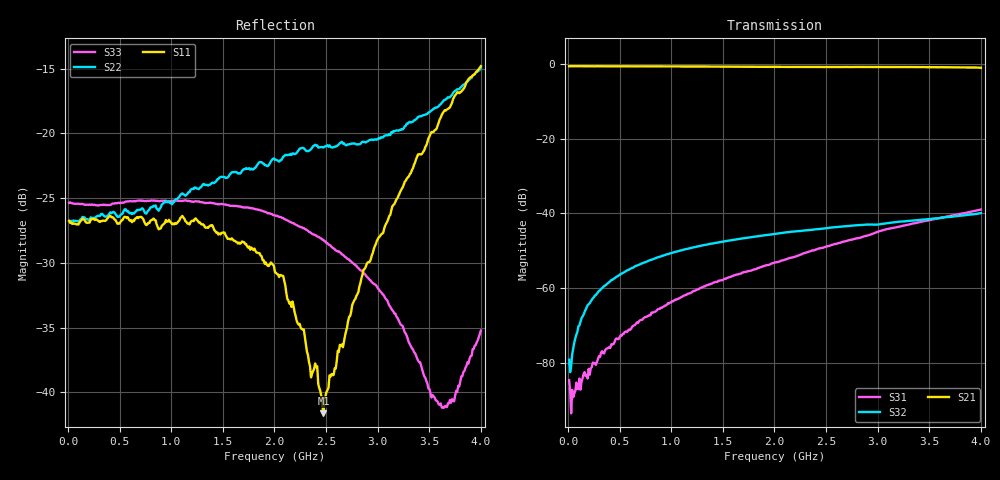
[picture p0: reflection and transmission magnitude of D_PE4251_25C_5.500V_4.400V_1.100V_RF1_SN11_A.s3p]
! Device ID: PE4251_SoldCshunt_081809
! Dir: c:\Test Bench Repositories\Bench_Software_CVI_Version_8\trunk\PSC 4Port_VNA Bench\datalog\4250\TEST\PE4251_SoldCshunt_081809\25C\5p500000\RF1
! Serial: 11
! Insertion: A
! Temp: 25C
! VDD: 5.500
! Control_Hi: 80.000
! Control_Lo: 20.000
! Logic State: RF1
! Port 1: RFC
! Port 2: RF1
! Port 3: RF2
! V1 = 1.10
! V2 = 4.40
! V3 = 1.10
! IDD: 6.772010e-05
! FILE NAME
! DATE 08/18/09  20:15
! CORRECTED  DATA
#  Hz  S  RI  R  50.00
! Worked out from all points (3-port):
!   401 points, 10 MHz to 4 GHz, reference 50 ohm
!   strongest paths, dB at 10 MHz, 1.008 GHz, 2.005 GHz, 3.002 GHz, 4 GHz:
!     S21: -0.6, -0.6, -0.7, -0.7, -1.0
!     S32: -79.2, -50.6, -45.5, -43.0, -39.9
!     S31: -84.7, -63.5, -53.1, -44.9, -39.0
!   lowest |S11| = -41.6 dB at 2.474 GHz (marker M1), VSWR 1.02, Z = 49.9 - j0.828 ohm
!   |S11| at or under -10 dB: start of sweep to end of sweep
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1e7  0.046 -4.05e-05  0.9371 -0.00367  3.37e-05 -4.18e-05
     0.9379 -0.00443  0.0459 5.96e-05  1.15e-05 1.23e-05
     -7.24e-06 -5.79e-05  0.000109 5.09e-06  0.0539 -0.000166
9.9775e7  0.0445 -0.000588  0.9389 -0.0344  2.22e-05 -3.6e-05
          0.9384 -0.0345  0.0457 -0.000485  4.19e-05 0.000299
          9.14e-06 -4.32e-05  3.49e-05 0.000305  0.0535 -0.000366
1.8955e8  0.0452 0.000221  0.9366 -0.0643  -5.5e-06 -7.37e-05
          0.9356 -0.064  0.0466 -0.000106  5.89e-05 0.000574
          1.03e-05 -6.05e-05  5.76e-05 0.000586  0.053 -0.000928
5.0875e8  0.0453 -0.00476  0.9205 -0.1672  -0.000149 -0.000168
          0.9209 -0.1668  0.0483 -0.00367  0.00015 0.00152
          -0.000153 -0.000175  0.000152 0.00153  0.0537 -0.00501
1.137175e9  0.0429 -0.0161  0.8588 -0.3606  -0.000771 -0.00025
            0.859 -0.3591  0.0548 -0.0175  0.000581 0.00326
            -0.000772 -0.000232  0.000574 0.00326  0.0547 -0.00713
2.005e9  0.0263 -0.0126  0.7173 -0.5776  -0.00218 -0.000168
         0.7173 -0.5775  0.0692 -0.0385  0.00109 0.0052
         -0.0022 -0.000166  0.00107 0.00521  0.048 -0.00412
2.473825e9  -0.000476 -0.00828  0.6241 -0.6729  -0.00347 -0.000169
            0.621 -0.6721  0.0635 -0.0613  0.00118 0.00614
            -0.00347 -0.000174  0.00118 0.00614  0.0388 -0.00012
2.872825e9  -0.0195 -0.0227  0.5309 -0.7485  -0.00494 1.57e-05
            0.5328 -0.7461  0.043 -0.0822  0.00123 0.00691
            -0.00495 -4.21e-06  0.00124 0.00693  0.0286 0.00266
3.62095e9  -0.098 -0.0656  0.3176 -0.8512  -0.00862 0.00164
           0.3188 -0.8523  -0.045 -0.1234  0.000236 0.00872
           -0.00864 0.00164  0.000244 0.00872  0.00208 0.00847
4e9  -0.1633 -0.0802  0.1852 -0.8778  -0.0108 0.00304
     0.1841 -0.8749  -0.1249 -0.1279  -0.000448 0.0101
     -0.0108 0.00305  -0.000485 0.0101  -0.014 0.0102
